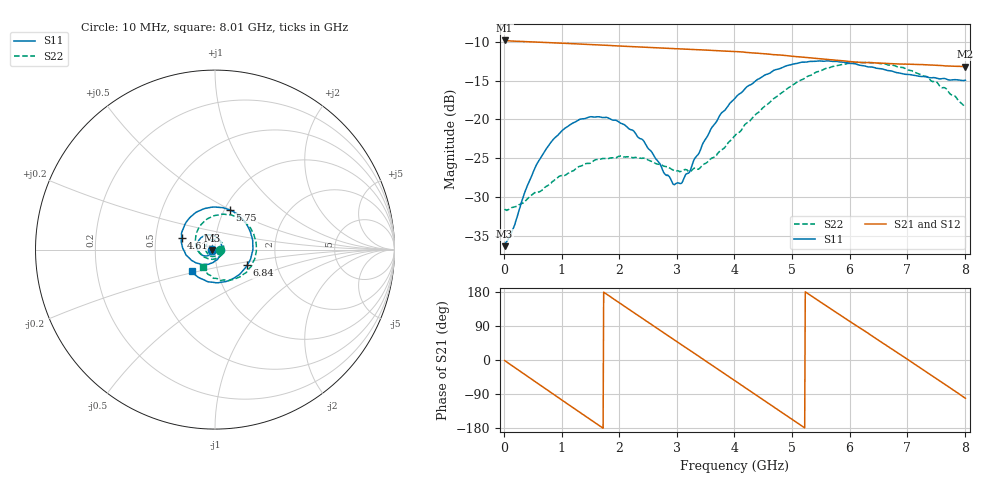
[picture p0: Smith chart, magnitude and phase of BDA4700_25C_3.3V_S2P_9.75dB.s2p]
!Agilent Technologies,E5071B,MY42404982,A.09.10
!Date: Mon Oct 20 18:07:06 2025
!Data & Calibration Information:
!Freq	S11:SOLT2(ON)	S21:SOLT2(ON)	S12:SOLT2(ON)	S22:SOLT2(ON)
# Hz S RI R 50
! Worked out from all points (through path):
!   801 points, 10 MHz to 8.01 GHz, reference 50 ohm
!   highest |S21| = -9.86 dB at 10 MHz (marker M1); lowest = -13.2 dB at 8.01 GHz (marker M2)
!   group delay of S21, straight-line fit = 284 ps
!   lowest |S11| = -36.2 dB at 10 MHz (marker M3), VSWR 1.03, Z = 48.5 - j0.129 ohm
!   |S11| at or under -10 dB: start of sweep to end of sweep
!   |S22| runs from -31.7 to -12.7 dB; largest |S21 - S12| = 0.0036
!   S11 on the Smith chart (normalised r, x): 10 MHz: 0.97, -0.00; 4.61 GHz: 0.68, +0.09; 5.75 GHz: 1.06, +0.50; 6.84 GHz: 1.41, -0.26; 8.01 GHz: 0.75, -0.19
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1e7  -0.0153 -0.00133  0.3212 -0.00699  0.3209 -0.00728  0.0266 -0.00134
3.3e8  -0.0228 -0.022  0.2586 -0.1823  0.2584 -0.1823  0.0225 -0.0184
7.2e8  -0.053 -0.0353  0.075 -0.3027  0.0751 -0.3025  0.000153 -0.0369
1.02e9  -0.0825 -0.0231  -0.0918 -0.2943  -0.0918 -0.2944  -0.0265 -0.0347
1.35e9  -0.1004 0.0112  -0.2387 -0.1888  -0.2386 -0.1891  -0.0498 -0.0083
1.64e9  -0.0923 0.0485  -0.2976 -0.0434  -0.2977 -0.0435  -0.0501 0.0238
1.93e9  -0.0632 0.0762  -0.276 0.1097  -0.276 0.1097  -0.0272 0.0496
2.32e9  -0.00953 0.0768  -0.1382 0.2572  -0.1382 0.2571  0.0169 0.0544
2.68e9  0.0308 0.0439  0.0433 0.2848  0.0428 0.2846  0.046 0.0235
2.94e9  0.0382 0.00404  0.1643 0.2329  0.164 0.2322  0.0469 -0.00624
3.08e9  0.0343 -0.0186  0.2164 0.1831  0.2145 0.1845  0.0407 -0.0226
3.53e9  -0.02 -0.0752  0.277 -0.027  0.2772 -0.0275  -0.00561 -0.0529
4.01e9  -0.1199 -0.0661  0.1567 -0.2232  0.1569 -0.2227  -0.0714 -0.0333
4.61e9  -0.1864 0.0666  -0.1181 -0.2341  -0.1175 -0.2347  -0.1074 0.0704
4.99e9  -0.1468 0.1707  -0.232 -0.1052  -0.2323 -0.1058  -0.0674 0.1499
5.35e9  -0.0501 0.2304  -0.242 0.0534  -0.2423 0.052  0.0181 0.1924
5.75e9  0.0829 0.2207  -0.1452 0.1912  -0.1447 0.1912  0.1332 0.1754
6.19e9  0.1874 0.1198  0.0265 0.2305  0.0294 0.2311  0.22 0.0727
6.68e9  0.2018 -0.0396  0.189 0.1284  0.1894 0.1281  0.2118 -0.0704
6.84e9  0.1792 -0.0875  0.2156 0.0712  0.216 0.0694  0.1868 -0.1098
7.33e9  0.0568 -0.1789  0.1913 -0.1167  0.1914 -0.117  0.0736 -0.1742
8.01e9  -0.1303 -0.122  -0.0418 -0.214  -0.041 -0.2143  -0.0675 -0.0986
